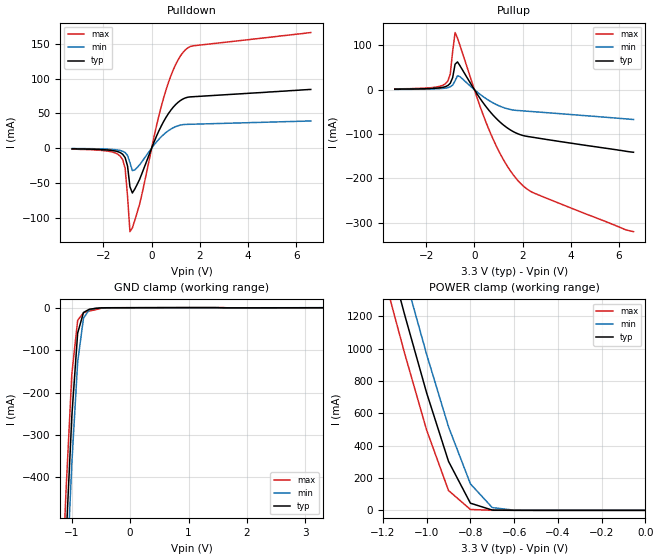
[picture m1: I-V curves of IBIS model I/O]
|   TEXAS INSTRUMENTS INCORPORATED
|   Standard Linear and Logic
|   IBIS Model of SN74ALVCH16901
|   18-BIT Universal Bus Transceiver with Parity Generators/Checkers
|   64-pin DGG Package
[IBIS Ver]   2.1
[Comment char]  |_char
[File Name]   alvch16901.ibs
[File Rev]   1.0
[Date]   04/10/98
[Source]   File originated at Texas Instruments, Inc.
[Notes]   The following is an IBIS list for the ALVCH16901.
|   - This file may be incomplete or may not be fully compliant
|   with the IBIS specification. It will be replaced with a
|   version that is IBIS Revision 3.2 compliant and is complete
|   and accurate.  Please email all questions and comments to
|   sllibis@ti.com.
|   - All test data contained in this file are derived from
|   hspice(tm) simulations.
|   - File created by David Yaeger, SLL Applications
[Disclaimer]
* Property of Texas Instruments Incorporated.  Unauthorized *
* reproduction and/or distribution is strictly prohibited. *
* This product is protected under copyright law. *
* Created 1997, (C) Copyright 1997, Texas Instruments Inc., *
* All Rights Reserved *
* UNLESS THERE IS A SIGNED, WRITTEN AGREEMENT TO THE *
* CONTRARY, TEXAS INSTRUMENTS ("TI") IS PROVIDING THE IBIS *
* MODELS "AS IS" AND WITHOUT ANY WARRANTY, EXPRESSED OR *
* IMPLIED.  TI assumes no liability for: *
* 1) the accuracy of the IBIS models provided to your *
* company; *
* 2) the proper functioning of these IBIS models in your *
* design or for any resulting applications; or *
* 3) infringement of patents, copyrights or intellectual *
* property rights resulting from your use of these *
* IBIS models. *
* TI provides IBIS Models as a service to our customers. *
* You and your company shall not distribute, sell or give *
* these models to anyone else without prior written *
* permission from TI. *
* TI reserves the right to make changes to our products or *
* to discontinue any semiconductor product or service *
* without notice, and advises our customers to obtain the *
* latest version of relevant information to verify, before *
* placing orders, that the information being relied on is *
* current. *
* Please be aware that your receipt and use of the IBIS *
* information provided shall serve as acceptance of these *
* terms and conditions.  If you do not accept these terms, *
* you should return or destroy the IBIS models and any *
* other accompanying information immediately. *
[Component]   ALVCH16901_DGG
[Manufacturer]  Texas Instruments, Inc.
[Package]
|   typ   min   max
R_pkg   0.068   0.046   0.094
L_pkg   3.798nH   2.565nH   5.991nH
C_pkg   0.564pF   0.297pF   1.022pF
[Pin]   signal_name   model_name   R_pin   L_pin   C_pin
1   1CLKENAB_BAR   NC   0.094   5.991nH   0.94pF
2   LEAB   NC   0.09   5.514nH   1.005pF
3   CLKAB   NC   0.092   5.261nH   0.912pF
4   1EERA_BAR   NC   0.092   4.891nH   0.805pF
5   1APAR   NC   0.085   4.561nH   0.702pF
6   GND   GND   0.084   4.247nH   0.597pF
7   1A1   I/O   0.08   3.933nH   0.534pF
8   1A2   I/O   0.077   3.622nH   0.523pF
9   1A3   I/O   0.05   3.372nH   0.483pF
10   VCC   POWER   0.048   3.139nH   0.415pF
11   1A4   I/O   0.049   3.042nH   0.397pF
12   1A5   I/O   0.051   2.941nH   0.384pF
13   1A6   I/O   0.05   2.8nH   0.355pF
14   GND   GND   0.052   2.711nH   0.335pF
15   1A7   I/O   0.051   2.589nH   0.314pF
16   1A8   I/O   0.055   2.604nH   0.303pF
17   2A1   I/O   0.055   2.597nH   0.302pF
18   2A2   I/O   0.052   2.605nH   0.315pF
19   GND   GND   0.051   2.694nH   0.334pF
20   2A3   I/O   0.05   2.772nH   0.352pF
21   2A4   I/O   0.048   2.864nH   0.372pF
22   2A5   I/O   0.049   2.982nH   0.392pF
23   VCC   POWER   0.049   3.129nH   0.413pF
24   2A6   I/O   0.046   3.263nH   0.48pF
25   2A7   I/O   0.077   3.592nH   0.542pF
26   2A8   I/O   0.081   3.923nH   0.557pF
27   GND   GND   0.086   4.252nH   0.614pF
28   2APAR   NC   0.085   4.525nH   0.714pF
29   2ERRA_BAR   NC   0.087   4.81nH   0.813pF
30   OEAB_BAR   NC   0.089   5.135nH   0.918pF
31   SEL_BAR   NC   0.09   5.486nH   1.019pF
32   2CLKENAB_BAR   NC   0.09   5.912nH   0.936pF
33   2CLKENBA_BAR   NC   0.087   5.926nH   0.931pF
34   ODD/EVEN_BAR   NC   0.087   5.496nH   1.004pF
35   OEBA_BAR   NC   0.087   5.124nH   0.902pF
36   2ERRB_BAR   NC   0.088   4.867nH   0.807pF
37   2BPAR   NC   0.086   4.514nH   0.707pF
38   GND   GND   0.085   4.206nH   0.605pF
39   2B8   I/O   0.089   3.929nH   0.537pF
40   2B7   I/O   0.079   3.584nH   0.528pF
41   2B6   I/O   0.048   3.299nH   0.481pF
42   VCC   POWER   0.048   3.101nH   0.409pF
43   2B5   I/O   0.048   2.969nH   0.388pF
44   2B4   I/O   0.048   2.855nH   0.369pF
45   2B3   I/O   0.049   2.766nH   0.349pF
46   GND   GND   0.051   2.696nH   0.331pF
47   2B2   I/O   0.052   2.638nH   0.315pF
48   2B1   I/O   0.053   2.565nH   0.297pF
49   1B8   I/O   0.052   2.574nH   0.299pF
50   1B7   I/O   0.051   2.617nH   0.313pF
51   GND   GND   0.05   2.666nH   0.329pF
52   1B6   I/O   0.05   2.769nH   0.35pF
53   1B5   I/O   0.049   2.909nH   0.378pF
54   1B4   I/O   0.048   2.993nH   0.39pF
55   VCC   POWER   0.049   3.176nH   0.416pF
56   1B3   I/O   0.048   3.295nH   0.483pF
57   1B2   I/O   0.079   3.569nH   0.536pF
58   1B1   I/O   0.082   3.908nH   0.547pF
59   GND   GND   0.086   4.238nH   0.613pF
60   1BPAR   NC   0.086   4.509nH   0.714pF
61   1ERRB_BAR   NC   0.089   4.863nH   0.822pF
62   CLKBA   NC   0.09   5.197nH   0.923pF
63   LEBA   NC   0.092   5.558nH   1.022pF
64   1CLKENBA_BAR   NC   0.09   5.947nH   0.946pF
| Models and submodels in the file (1): I/O (I/O)
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|   Model ALVCH16901_I/O
[Model]   I/O
Model_type   I/O
Polarity   Non-Inverting
Enable   Active-Low
Vinl = 0.8V
Vinh = 2.0V
|Variable   typ   min   max
C_comp   7.0pF   NA   NA
[Voltage range]   3.3   3.0   3.6
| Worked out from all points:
|   slope of the pulldown table from 0 to 0.495 V, typ, clamps not added: 12.9 ohm
|   slope of the pullup table from 0 to 0.495 V, typ, clamps not added: 12.6 ohm
|   GND clamp passes 1 mA (typ) near -0.54 V on its own axis
|   POWER clamp passes 1 mA (typ) near -0.65 V on its own axis
[Pullup]   | Note: Vtable = Vcc - Voutput
|   Voltage   I(typ)   I(min)   I(max)
-3.3V     1mA        600uA      1.6mA
-1.2V     6.7mA      3.4mA      13.3mA
-1V       14.29mA    6.322mA    35.01mA
-900mV    27.23mA    10.23mA    86.35mA
-800mV    57.41mA    19.92mA    128.7mA
-700mV    62.45mA    31.18mA    116.2mA
-600mV    54.15mA    29.3mA     100.1mA
600mV     -46.39mA   -24.34mA   -89.47mA
1.2V      -79.51mA   -40.29mA   -157.5mA
1.8V      -99.5mA    -47.06mA   -204.7mA
2.5V      -108.1mA   -49.91mA   -233.8mA
6.6V      -141.2mA   -67.3mA    -320.2mA
[Pulldown]
|   Voltage   I(typ)   I(min)   I(max)
-3.3V     -1mA       -600uA     -1.6mA
-1.3V     -6.5mA     -3.4mA     -11.6mA
-1.1V     -13.6mA    -6.415mA   -29.06mA
-1V       -25.75mA   -10.55mA   -69.33mA
-900mV    -55.74mA   -20.99mA   -120.4mA
-800mV    -64.66mA   -32.41mA   -115mA
-700mV    -59.03mA   -31.35mA   -104.3mA
500mV     38.59mA    19.72mA    72.79mA
900mV     59.2mA     29.44mA    113.2mA
1.3V      70.86mA    33.89mA    137.9mA
1.7V      74.07mA    34.47mA    147.4mA
6.6V      84.6mA     39.1mA     166.6mA
[POWER_Clamp]   | Note: Vtable = Vcc - Voutput
|   Voltage   I(typ)   I(min)   I(max)
-3.3V     13.16A     13.37A     12.95A
-1.2V     1.713A     1.957A     1.472A
-1.1V     1.207A     1.451A     967.8mA
-1V       726.3mA    964.5mA    496.3mA
-900mV    302.9mA    516.9mA    122.7mA
-800mV    44.4mA     164.1mA    5.51mA
-700mV    1.811mA    17.06mA    344.6uA
-600mV    194.7uA    1.012mA    215.5uA
0V        1.787nA    1.691nA    1.867nA
[GND_Clamp]
|   Voltage   I(typ)   I(min)   I(max)
-3.3V     -8.62A     -8.72A     -8.526A
-1.2V     -880mA     -1.002A    -761.7mA
-1.1V     -550.7mA   -671.6mA   -434.3mA
-1V       -256.1mA   -367.6mA   -156.7mA
-900mV    -59.85mA   -128.1mA   -29.79mA
-800mV    -11.26mA   -24.35mA   -11.83mA
-700mV    -3.568mA   -4.883mA   -7.7mA
-600mV    -1.845mA   -1.247mA   -4.967mA
-400mV    -104uA     -65.92uA   -148.3uA
3.3V      1.785nA    46.78uA    -102.1uA
[Ramp]
| variable   typ   min   max
dV/dt_r   1.5710E+00/2.8906E-10  1.1583E+00/5.4169E-10  1.9146E+00/1.5046E-10
dV/dt_f   1.5583E+00/3.6661E-10  1.0744E+00/9.3999E-10  1.9079E+00/1.8103E-10
